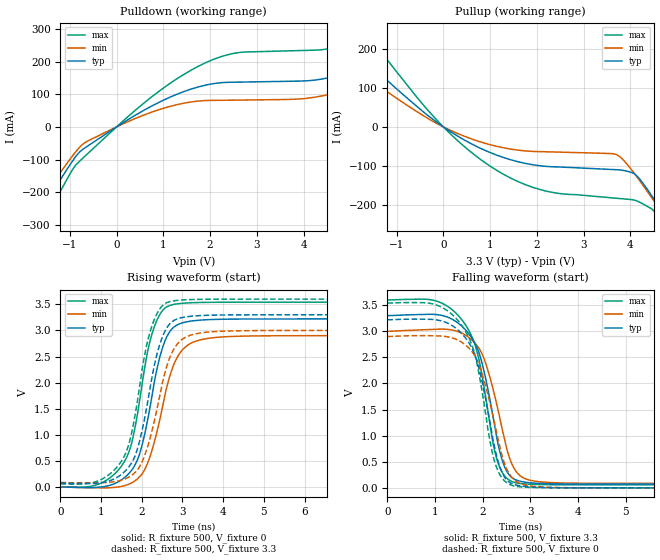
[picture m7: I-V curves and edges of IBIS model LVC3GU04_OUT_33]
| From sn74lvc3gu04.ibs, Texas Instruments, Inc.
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[Model]   LVC3GU04_OUT_33
Model_type  Output
Vref =   0
Rref =   500
Cref =   50p
Vmeas =   1.5
| variable   typ   min   max
C_comp   11.31pF   6.54pF   15.99pF
| C_pullup   12.43pF   6.68pF   15.99pF
| C_pulldown   10.19pF   6.54pF   14.34pF
[Temperature Range]   40   100   -40
| Ambient temperature   25   85   -40
[Voltage range]   3.3   3   3.6
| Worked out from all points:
|   slope of the pulldown table from 0 to 0.495 V, typ, clamps not added: 11.4 ohm
|   slope of the pullup table from 0 to 0.495 V, typ, clamps not added: 13.6 ohm
|   rising waveform, R_fixture 500, V_fixture 0: 20-80 % time 524ps typ, 574ps min, 516ps max; typ from 0 V to 3.22 V
|   falling waveform, R_fixture 500, V_fixture 3.3: 20-80 % time 459ps typ, 478ps min, 463ps max; typ from 3.3 V to 0.072 V
|   rising waveform, R_fixture 500, V_fixture 3.3: 20-80 % time 525ps typ, 559ps min, 515ps max; typ from 0.072 V to 3.3 V
|   falling waveform, R_fixture 500, V_fixture 0: 20-80 % time 460ps typ, 481ps min, 463ps max; typ from 3.22 V to 0 V
[Pulldown]
| LVC3GU04_OUT_33
|   Voltage   I(typ)   I(min)   I(max)
-5.5V     -1.112A    -993.8mA   -1.301A
-2.14V    -375.5mA   -330.4mA   -447.6mA
-1.44V    -215.5mA   -187.5mA   -260.6mA
-925mV    -101.1mA   -85.57mA   -127mA
-610mV    -57.74mA   -42.74mA   -80.75mA
1.115V    89.28mA    61.7mA     130.4mA
2.37V     136.6mA    81.79mA    220.7mA
4.9V      164.6mA    112.8mA    253.7mA
5.705V    210.7mA    154.2mA    308.6mA
6.855V    302.8mA    233.5mA    425.8mA
7.69V     383.3mA    301.9mA    530.5mA
11V       772.7mA    631.3mA    1.042A
[Pullup]
| LVC3GU04_OUT_33
|   Voltage   I(typ)   I(min)   I(max)
-5.5V     658.4mA    524.1mA    915.7mA
-2.975V   326.7mA    254.3mA    462mA
-2.255V   238.9mA    184.2mA    340.3mA
-1.835V   189.7mA    145.3mA    271.6mA
-90mV     7.531mA    5.5mA      11.13mA
1.035V    -67.22mA   -46.55mA   -103.1mA
2.18V     -100.8mA   -63.53mA   -163.7mA
3.695V    -109.4mA   -70.5mA    -182.4mA
4.12V     -123.3mA   -124.6mA   -188.6mA
4.715V    -223.6mA   -226.6mA   -253mA
4.885V    -255.9mA   -257.1mA   -287.8mA
11V       -1.523A    -1.428A    -1.712A
[Ramp]
| LVC3GU04_OUT_33
| variable   typ   min   max
dV/dt_r   1.94/5.34E-10   1.75/5.83E-10   2.13/5.22E-10
dV/dt_f   1.95/4.74E-10   1.77/4.92E-10   2.14/4.76E-10
R_load = 500
[Rising Waveform]
| LVC3GU04_OUT_33
R_fixture =   500
C_fixture =   0
L_fixture =   0
V_fixture =   0
V_fixture_min = 0
V_fixture_max = 0
|   Time   V(typ)   V(min)   V(max)
0s        386.6pV    4.76nV     2.624uV
1.145ns   16.83mV    -18mV      135mV
1.765ns   337.2mV    84.72mV    887.9mV
1.995ns   767.2mV    237.3mV    1.905V
2.27ns    1.835V     753.9mV    2.983V
2.525ns   2.704V     1.594V     3.395V
2.81ns    3.077V     2.388V     3.502V
3.275ns   3.186V     2.779V     3.533V
4.355ns   3.218V     2.888V     3.541V
24.99ns   3.22V      2.9V       3.541V
[Falling Waveform]
| LVC3GU04_OUT_33
R_fixture =   500
C_fixture =   0
L_fixture =   0
V_fixture =   3.3
V_fixture_min = 3
V_fixture_max = 3.6
|   Time   V(typ)   V(min)   V(max)
0s        3.3V       3V         3.6V
1.025ns   3.321V     3.039V     3.581V
1.61ns    3.058V     2.942V     3.164V
1.955ns   2.498V     2.624V     2.315V
2.21ns    1.406V     1.923V     891.7mV
2.32ns    854.4mV    1.504V     488.5mV
2.49ns    345.7mV    812.3mV    199.9mV
2.72ns    144.8mV    292.8mV    92.12mV
3.965ns   73.37mV    89.11mV    58.41mV
24.99ns   72.43mV    85.87mV    58.1mV
[Rising Waveform]
| LVC3GU04_OUT_33
R_fixture =   500
C_fixture =   0
L_fixture =   0
V_fixture =   3.3
V_fixture_min = 3
V_fixture_max = 3.6
|   Time   V(typ)   V(min)   V(max)
0s        72.43mV    85.87mV    58.1mV
1.12ns    99.56mV    84.38mV    194.4mV
1.715ns   418.9mV    203.6mV    919mV
1.955ns   908.2mV    400.5mV    1.966V
2.23ns    2.015V     1.014V     3.042V
2.48ns    2.819V     1.893V     3.451V
2.77ns    3.181V     2.618V     3.565V
3.2ns     3.271V     2.91V      3.591V
4.24ns    3.298V     2.991V     3.6V
24.99ns   3.3V       3V         3.6V
[Falling Waveform]
| LVC3GU04_OUT_33
R_fixture =   500
C_fixture =   0
L_fixture =   0
V_fixture =   0
V_fixture_min = 0
V_fixture_max = 0
|   Time   V(typ)   V(min)   V(max)
0s        3.22V      2.9V       3.541V
995ps     3.223V     2.914V     3.515V
1.56ns    2.959V     2.792V     3.115V
1.76ns    2.702V     2.628V     2.769V
1.895ns   2.381V     2.42V      2.318V
2.145ns   1.303V     1.659V     940.7mV
2.27ns    701.8mV    1.159V     447.1mV
2.475ns   186.4mV    428.7mV    120mV
2.695ns   56.92mV    129.5mV    29.25mV
24.99ns   3.674nV    10.86nV    2.626uV
